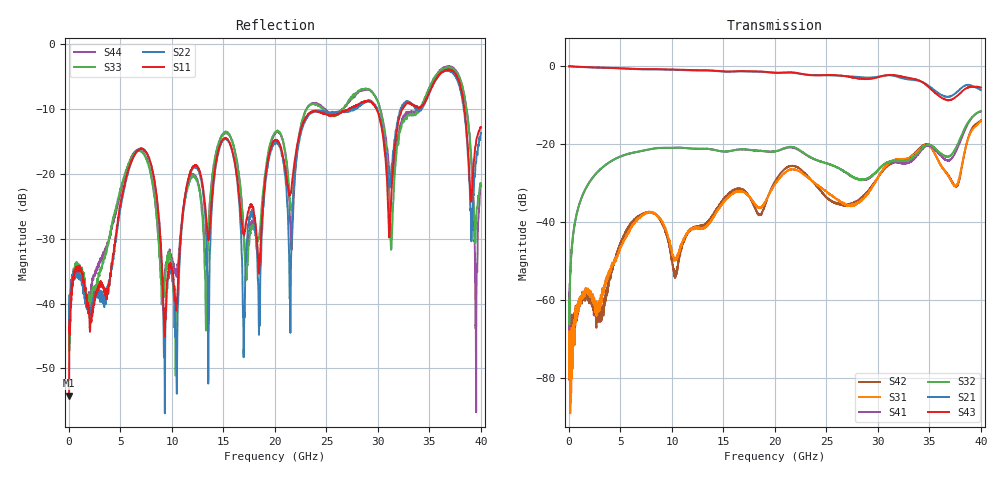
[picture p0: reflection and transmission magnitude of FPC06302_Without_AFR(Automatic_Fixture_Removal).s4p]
!The following data was pulled from an Agilent PNA
!This sNp file was generated from the data in the RF Test software
!NOTE:  Smoothing/Math/Corrections applied on any given trace ARE included in the data saved here
# MHz S dB R 50
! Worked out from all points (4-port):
!   4000 points, 10 MHz to 40 GHz, reference 50 ohm
!   strongest paths, dB at 10 MHz, 10.01 GHz, 20.01 GHz, 30.01 GHz, 40 GHz:
!     S43: 0.0, -0.9, -1.7, -2.9, -5.5
!     S21: -0.1, -0.9, -1.7, -2.7, -6.2
!     S32: -59.8, -21.0, -21.9, -26.7, -11.6
!     S41: -61.1, -21.0, -21.9, -26.7, -11.7
!     S31: -63.3, -47.9, -30.3, -28.5, -13.9
!     S42: -60.1, -49.9, -29.6, -28.5, -13.9
!   lowest |S11| = -54.2 dB at 10 MHz (marker M1), VSWR 1.00, Z = 50.2 - j0.0497 ohm
!   |S11| at or under -10 dB: start of sweep to 27.17 GHz; 29.84 GHz to 32.39 GHz (2.544 GHz wide, 8.18 % of centre); 38.41 GHz to end of sweep
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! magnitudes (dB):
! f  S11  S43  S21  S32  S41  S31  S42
! 10 MHz  -54.2  0.0  -0.1  -59.8  -61.1  -63.3  -60.1
! 4.65 GHz  -28.2  -0.5  -0.6  -23.6  -23.6  -48.9  -48.0
! 10.39 GHz  -40.6  -0.9  -1.0  -20.9  -21.0  -49.4  -52.6
! 12.03 GHz  -18.9  -1.0  -1.1  -21.2  -21.2  -41.6  -41.9
! 17 GHz  -29.5  -1.3  -1.4  -21.3  -21.4  -32.4  -31.9
! 36.84 GHz  -3.9  -8.8  -7.9  -23.2  -24.2  -28.3  -28.1
! 40 GHz  -12.9  -5.5  -6.2  -11.6  -11.7  -13.9  -13.9
